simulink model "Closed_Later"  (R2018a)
settings: Solver=ode45  StartTime=0.0  StopTime=20  RelTol=1e-3  EnableMultiTasking=on
StartFcn:
  | init
StopFcn:
  | pl
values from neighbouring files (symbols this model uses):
  Aact = [0, 1; -omg^2, -2*zet*omg]    [init.m]
  Bact = [0; omg^2]    [init.m]
  Cact = [1,0]    [init.m]
  Cyb = -0.0245    [init.m]    (also in lqr_des.m)
  Cydel = [-0.24668,0.24668, 0.47413,-0.47413,0]/100    [init.m]    (also in lqr_des.m = [-0.24668,0.24668, 0.47413,-0.47413]/100)
  d2r = pi/180    (= 0.0174532925199)    [init.m]
  Dact = 0    [init.m]
  Mass = 198.32    [init.m]    (also in lqr_des.m)
  Qbar = 150    [init.m]    (also in lqr_des.m)
  r2d = 180/pi    (= 57.2957795131)    [init.m]    (also in pl.m)
  Sref = 79.069    [init.m]    (also in lqr_des.m)
undefined symbols (not defined in the file or in its folder): Ap, Bp, Cp, Dp, Kmix, Kpr

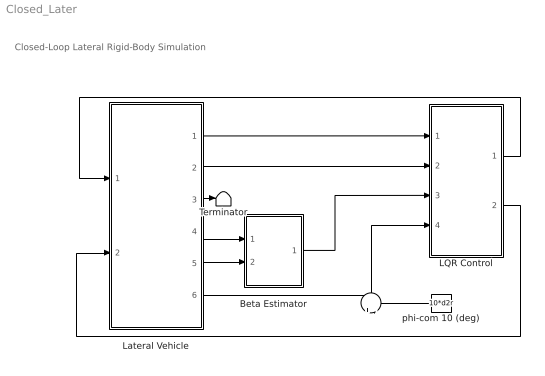
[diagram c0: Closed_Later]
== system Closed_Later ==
  note: Closed-Loop Lateral Rigid-Body Simulation
  " " : Sum  Inputs=+|-
  Beta Estimator : Subsystem
  LQR Control : Subsystem
  Lateral Vehicle : Subsystem
  Terminator : Terminator
  phi-com 10 (deg) : Constant  Value=10*d2r
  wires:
  LQR Control/2(dR) -> Lateral Vehicle/2(dR)
  LQR Control/1(dP) -> Lateral Vehicle/1(dP)
  Lateral Vehicle/1(p) -> LQR Control/1(p)
  Lateral Vehicle/2(r) -> LQR Control/2(r)
  Lateral Vehicle/5(Ny) -> Beta Estimator/2(Ydd)
  Lateral Vehicle/4(delta) -> Beta Estimator/1(delta)
  Beta Estimator/1(beth) -> LQR Control/3(beta)
  phi-com 10 (deg)/1 -> " "/2
  Lateral Vehicle/3(beta) -> Terminator/1
  Lateral Vehicle/6(phi) -> " "/1
  " "/1 -> LQR Control/4(phi)

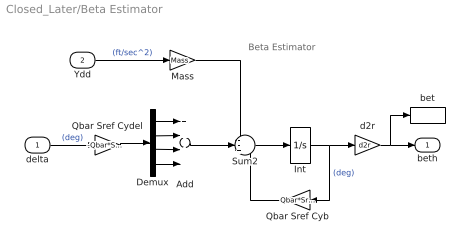
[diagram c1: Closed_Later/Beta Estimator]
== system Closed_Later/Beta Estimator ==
  note: Beta Estimator
  delta : Inport
  Ydd : Inport  Port=2
  Add : Sum  Inputs=++++
  Demux : Demux
  Int : Integrator
  Mass : Gain  Gain=Mass
  Qbar Sref Cyb : Gain  Gain=Qbar*Sref*Cyb
  Qbar Sref Cydel : Gain  Gain=-Qbar*Sref*Cydel
  Sum2 : Sum  Inputs=--+
  bet : ToWorkspace  VariableName=bethat  SampleTime=-1
  d2r : Gain  Gain=d2r
  beth : Outport
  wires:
  Demux/4 -> Add/4
  Demux/3 -> Add/3
  Demux/2 -> Add/2
  Demux/1 -> Add/1
  Qbar Sref Cydel/1 -> Demux/1
  delta/1 -> Qbar Sref Cydel/1  "(deg)"
  Sum2/1 -> Int/1
  Int/1 -> d2r/1, Qbar Sref Cyb/1  "(deg)"
  Qbar Sref Cyb/1 -> Sum2/3
  Ydd/1 -> Mass/1  "(ft/sec^2)"
  Mass/1 -> Sum2/1
  d2r/1 -> beth/1, bet/1
  Add/1 -> Sum2/2

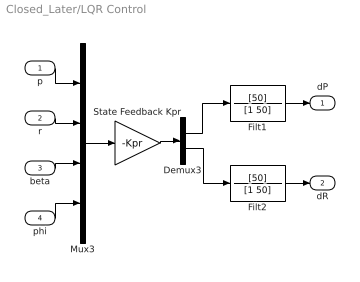
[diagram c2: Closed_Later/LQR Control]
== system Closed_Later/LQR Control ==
  p : Inport
  r : Inport  Port=2
  beta : Inport  Port=3
  phi : Inport  Port=4
  Demux3 : Demux  Outputs=2
  Filt1 : TransferFcn  Numerator=[50]  Denominator=[1 50]
  Filt2 : TransferFcn  Numerator=[50]  Denominator=[1 50]
  Mux3 : Mux
  State Feedback Kpr : Gain  Gain=-Kpr  Multiplication=Matrix(K*u) (u vector)
  dP : Outport
  dR : Outport  Port=2
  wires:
  State Feedback Kpr/1 -> Demux3/1
  Mux3/1 -> State Feedback Kpr/1
  p/1 -> Mux3/1
  r/1 -> Mux3/2
  Demux3/1 -> Filt1/1
  beta/1 -> Mux3/3
  phi/1 -> Mux3/4
  Demux3/2 -> Filt2/1
  Filt1/1 -> dP/1
  Filt2/1 -> dR/1

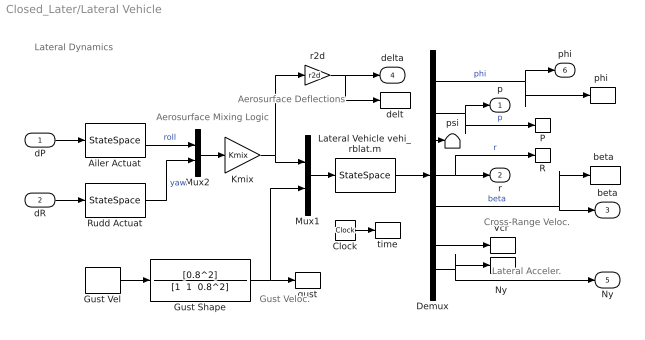
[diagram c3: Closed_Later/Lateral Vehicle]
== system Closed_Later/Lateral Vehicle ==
  note: Aerosurface Deflections
  note: Lateral Dynamics
  note: Aerosurface Mixing Logic
  note: Gust Veloc.
  note: Lateral Acceler.
  note: Cross-Range Veloc.
  dP : Inport
  dR : Inport  Port=2
  Ailer Actuat : StateSpace  A=Aact  B=Bact  C=Cact  D=Dact  InitialCondition=0
  Clock : Clock
  Demux : Demux  Outputs=7
  Gust Shape : TransferFcn  Numerator=[0.8^2]  Denominator="[1  1  0.8^2]"
  Gust Vel : DiscretePulseGenerator  PulseType=Time based  Amplitude=90  Period=35  PulseWidth=4  PhaseDelay=5
  Kmix : Gain  Gain=Kmix  Multiplication=Matrix(K*u) (u vector)
  Lateral Vehicle vehi_rblat.m : StateSpace  A=Ap  B=Bp  C=Cp  D=Dp  InitialCondition=0
  Mux1 : Mux  Inputs=[4,1]
  Mux2 : Mux  Inputs=2
  "Ny " : ToWorkspace  VariableName=Ny  SampleTime=-1
  P : ToWorkspace  VariableName=p  SampleTime=-1
  R : ToWorkspace  VariableName=r  SampleTime=-1
  Rudd Actuat : StateSpace  A=Aact  B=Bact  C=Cact  D=Dact  InitialCondition=0
  "Vcr " : ToWorkspace  VariableName=Vcr  SampleTime=-1
  "beta " : ToWorkspace  VariableName=beta  SampleTime=-1
  delt : ToWorkspace  VariableName=delta  SampleTime=-1
  gust : ToWorkspace  VariableName=gust  SampleTime=-1
  "phi " : ToWorkspace  VariableName=phi  SampleTime=-1
  psi : Terminator
  r2d : Gain  Gain=r2d
  time : ToWorkspace  VariableName=time  SampleTime=-1
  p : Outport
  r : Outport  Port=2
  beta : Outport  Port=3
  delta : Outport  Port=4
  Ny : Outport  Port=5
  phi : Outport  Port=6
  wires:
  Mux1/1 -> Lateral Vehicle vehi_rblat.m/1
  Gust Vel/1 -> Gust Shape/1
  Kmix/1 -> Mux1/1, r2d/1
  Mux2/1 -> Kmix/1
  Rudd Actuat/1 -> Mux2/2  "yaw"
  Ailer Actuat/1 -> Mux2/1  "roll"
  Lateral Vehicle vehi_rblat.m/1 -> Demux/1
  Demux/5 -> beta/1, "beta "/1  "beta"
  Demux/1 -> phi/1, "phi "/1  "phi"
  Demux/2 -> p/1, P/1  "p"
  dP/1 -> Ailer Actuat/1
  Demux/4 -> r/1, R/1  "r"
  dR/1 -> Rudd Actuat/1
  Demux/6 -> "Vcr "/1
  Demux/7 -> "Ny "/1, Ny/1
  Gust Shape/1 -> Mux1/2, gust/1
  r2d/1 -> delta/1, delt/1
  Clock/1 -> time/1
  Demux/3 -> psi/1
